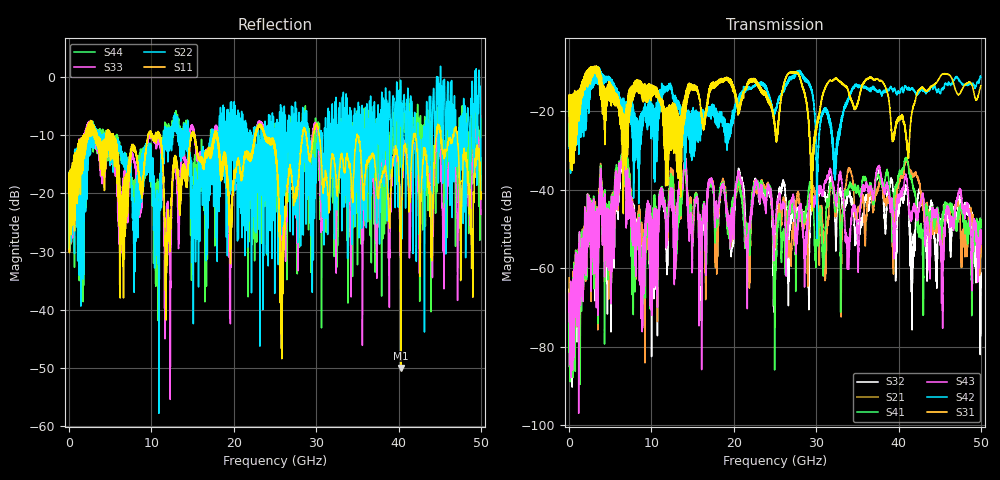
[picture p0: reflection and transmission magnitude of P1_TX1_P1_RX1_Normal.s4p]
!Keysight Technologies,N5225B,MY57041031,A.13.20.10
!Date: Friday, May 31, 2019 11:13:41
!Correction: S11(Full 4 Port(1,2,3,4))
!S12(Full 4 Port(1,2,3,4))
!S13(Full 4 Port(1,2,3,4))
!S14(Full 4 Port(1,2,3,4))
!S21(Full 4 Port(1,2,3,4))
!S22(Full 4 Port(1,2,3,4))
!S23(Full 4 Port(1,2,3,4))
!S24(Full 4 Port(1,2,3,4))
!S31(Full 4 Port(1,2,3,4))
!S32(Full 4 Port(1,2,3,4))
!S33(Full 4 Port(1,2,3,4))
!S34(Full 4 Port(1,2,3,4))
!S41(Full 4 Port(1,2,3,4))
!S42(Full 4 Port(1,2,3,4))
!S43(Full 4 Port(1,2,3,4))
!S44(Full 4 Port(1,2,3,4))
!S4P File: Measurements: <S11,S12,S13,S14>,
!<S21,S22,S23,S24>,
!<S31,S32,S33,S34>,
!<S41,S42,S43,S44>:
# Hz S  dB  R 50.0
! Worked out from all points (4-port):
!   5000 points, 10 MHz to 50 GHz, reference 50 ohm
!   strongest paths, dB at 10 MHz, 12.51 GHz, 25.01 GHz, 37.51 GHz, 50 GHz:
!     S31: -19.4, -29.2, -24.5, -11.8, -13.5
!     S42: -19.6, -14.8, -19.9, -15.1, -11.3
!     S43: -66.4, -41.8, -49.7, -34.3, -51.3
!     S41: -69.5, -38.7, -74.9, -36.4, -47.8
!     S21: -62.5, -36.7, -54.9, -40.0, -55.8
!     S32: -65.5, -39.6, -56.5, -36.9, -64.9
!   lowest |S11| = -50.0 dB at 40.27 GHz (marker M1), VSWR 1.01, Z = 49.7 - j0.0944 ohm
!   |S11| at or under -10 dB: 18.01 GHz to 22.61 GHz (4.595 GHz wide, 22.6 % of centre); 30.38 GHz to 34.94 GHz (4.562 GHz wide, 14 % of centre); 34.98 GHz to 41.81 GHz (6.838 GHz wide, 17.8 % of centre)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
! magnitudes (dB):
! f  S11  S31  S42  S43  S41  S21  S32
! 10 MHz  -19.9  -19.4  -19.6  -66.4  -69.5  -62.5  -65.5
! 6.53 GHz  -21.9  -24.6  -16.7  -30.8  -31.2  -31.6  -31.1
! 8.92 GHz  -19.6  -17.3  -20.1  -63.7  -58.1  -52.9  -56.9
! 14.05 GHz  -15.4  -18.7  -24.9  -33.2  -34.5  -34.4  -32.9
! 25.02 GHz  -12.6  -25.2  -19.4  -49.1  -65.3  -53.1  -55.2
! 40.27 GHz  -50.0  -21.3  -14.6  -41.2  -35.3  -36.3  -41.0
! 50 GHz  -19.8  -13.5  -11.3  -51.3  -47.8  -55.8  -64.9
